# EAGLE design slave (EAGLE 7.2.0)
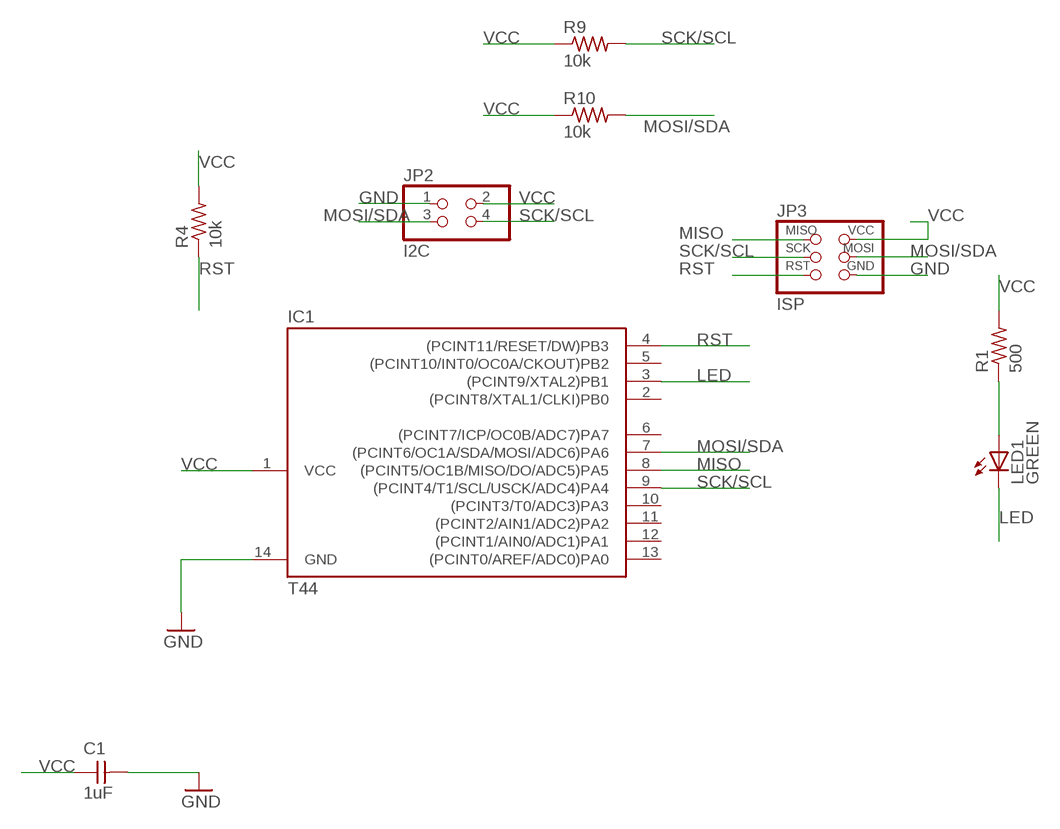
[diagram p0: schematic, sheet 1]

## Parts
C1  1uF  CAP-UNPOLARIZEDFAB  [C1206FAB]
IC1  T44  ATTINY44-SSU  [SOIC14]
JP2  I2C  PINHD-2X2-SMD  [2X02SMD]
JP3  ISP  AVRISPSMD  [2X03SMD]
LED1  GREEN  LEDFAB1206  [LED1206FAB]
R1  500  RES-US1206FAB  [R1206FAB]
R4  10k  RES-US1206FAB  [R1206FAB]
R9  10k  RES-US1206FAB  [R1206FAB]
R10  10k  RES-US1206FAB  [R1206FAB]

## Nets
GND: C1.2 IC1.14(GND) JP2.1 JP3.6(GND)
LED: IC1.3((PCINT9/XTAL2)PB1) LED1.2(C)
MISO: IC1.8((PCINT5/OC1B/MISO/DO/ADC5)PA5) JP3.1(MISO)
MOSI/SDA: IC1.7((PCINT6/OC1A/SDA/MOSI/ADC6)PA6) JP2.3 JP3.4(MOSI) R10.2
N$2: LED1.1(A) R1.1
RST: IC1.4((PCINT11/RESET/DW)PB3) JP3.5(RST) R4.1
SCK/SCL: IC1.9((PCINT4/T1/SCL/USCK/ADC4)PA4) JP2.4 JP3.3(SCK) R9.2
VCC: C1.1 IC1.1(VCC) JP2.2 JP3.2(VCC) R1.2 R4.2 R9.1 R10.1
Unconnected: IC1.2((PCINT8/XTAL1/CLKI)PB0) IC1.5((PCINT10/INT0/OC0A/CKOUT)PB2) IC1.6((PCINT7/ICP/OC0B/ADC7)PA7) IC1.10((PCINT3/T0/ADC3)PA3) IC1.11((PCINT2/AIN1/ADC2)PA2) IC1.12((PCINT1/AIN0/ADC1)PA1) IC1.13((PCINT0/AREF/ADC0)PA0)

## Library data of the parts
C1 = 02fab:CAP-UNPOLARIZED
IC1 = 02fab:ATTINY44
JP2 = 02fab:PINHD-2X2-SMD
JP3 = 02fab:AVRISP
LED1 = 02fab:LED: LED
R1 R4 R9 R10 = 02fab:RES-US: Resistor (US Symbol)

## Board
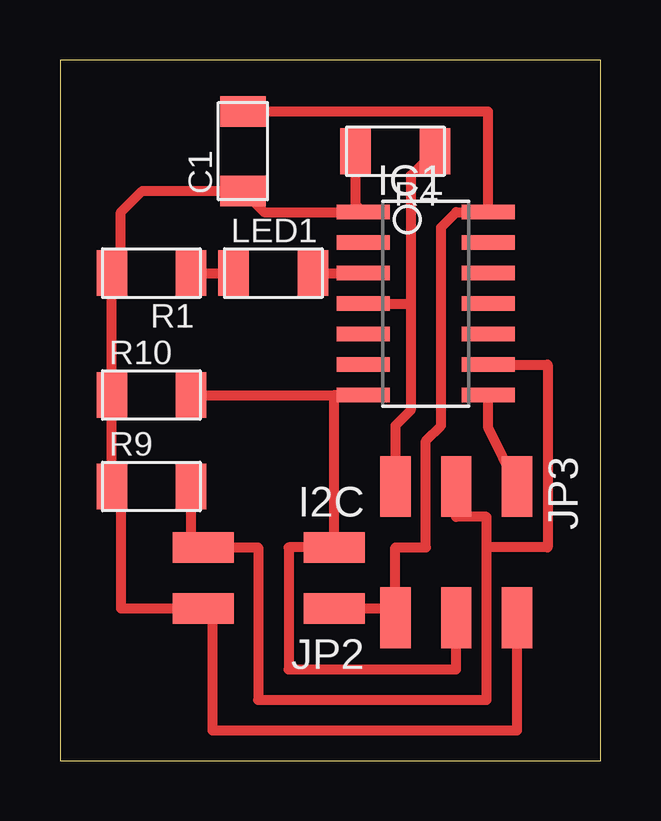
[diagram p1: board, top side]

Size 22.53 x 29.2 mm. Coordinates in mm from the lower left corner, seen from the top.
Outline: 0,0 22.53,0 22.53,29.2 0,29.2 0,0
Copper layers (1*16): Top 0.035mm / dielectric 1.5mm / Bottom 0.035mm
Design rules "default": minimum track width 10mil, minimum drill 24mil, track to track 8mil, track to pad 8mil, pad to pad 8mil, via to via 8mil, smd to smd 8mil, copper to edge 40mil, drill to drill 8mil, minimum pad ring 10mil, minimum via ring 8mil, stop-mask expansion 4mil, vias tented up to drill 0mil, thermal gap 10mil

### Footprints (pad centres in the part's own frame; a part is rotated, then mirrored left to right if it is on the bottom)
C1206FAB = smd 1.27 x 1.905: 1 -1.651,0; 2 1.651,0
SOIC14 = smd 0.61 x 2.21: 1 -3.81,-2.603; 2 -2.54,-2.603; 3 -1.27,-2.603; 4 0,-2.603; 5 1.27,-2.603; 6 2.54,-2.603; 7 3.81,-2.603; 8 3.81,2.603; 9 2.54,2.603; 10 1.27,2.603; 11 0,2.603; 12 -1.27,2.603; 13 -2.54,2.603; 14 -3.81,2.603
2X02SMD = smd 2.54 x 1.27: 1 -2.54,1.27; 2 2.92,1.27; 3 -2.54,-1.27; 4 2.92,-1.27
2X03SMD = smd 2.54 x 1.27: 1 -2.54,2.54; 2 2.92,2.54; 3 -2.54,0; 4 2.92,0; 5 -2.54,-2.54; 6 2.92,-2.54
LED1206FAB = smd 1.27 x 1.905: 1 -1.651,0; 2 1.651,0
R1206FAB = smd 1.27 x 1.905: 1 -1.651,0; 2 1.651,0

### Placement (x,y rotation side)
C1  7.62,25.4 90 top
IC1  15.24,19.05 270 top
JP2  8.89,7.62 180 top
JP3  16.51,8.89 270 top
LED1  8.89,20.32 0 top
R1  3.81,20.32 180 top
R4  13.97,25.4 180 top
R9  3.81,11.43 0 top
R10  3.81,15.24 0 top

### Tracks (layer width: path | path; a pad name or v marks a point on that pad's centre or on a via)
GND
  Top 0.406: IC1.14 17.78,22.86 | 13.97,6.35 JP3.6 13.97,5.08 | 13.97,6.35 13.97,8.89 15.24,8.89 15.24,13.34 15.88,13.97 15.88,22.23 16.51,22.86 IC1.14 | JP2.1 13.97,6.35 | IC1.14 17.84,27.05 C1.2
LED
  Top 0.406: LED1.2 IC1.3
MISO
  Top 0.406: JP3.1 17.84,13.91 IC1.8
MOSI/SDA
  Top 0.406: R10.2 11.43,15.24 | 11.43,15.24 IC1.7 | 11.43,15.24 JP2.3 9.53,8.89 9.53,3.81 16.51,3.81 JP3.4 16.51,6.35
N$2
  Top 0.406: R1.1 LED1.1
RST
  Top 0.406: R4.1 14.61,24.38 14.61,19.05 | IC1.4 14.61,19.05 | 14.61,19.05 14.61,14.61 13.97,13.97 JP3.5
SCK/SCL
  Top 0.406: R9.2 5.46,8.89 JP2.4 8.26,8.89 8.26,2.54 17.78,2.54 17.78,8.89 | 17.78,8.89 17.78,10.16 16.51,10.16 JP3.3 | IC1.9 20.32,16.51 20.32,8.89 17.78,8.89
VCC
  Top 0.406: R4.2 12.32,23.18 IC1.1 8.51,22.86 C1.1 3.43,23.75 2.54,22.86 2.54,20.7 R1.2 R10.1 R9.1 2.54,11.43 2.54,6.35 JP2.2 6.35,6.35 6.35,1.27 19.05,1.27 JP3.2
